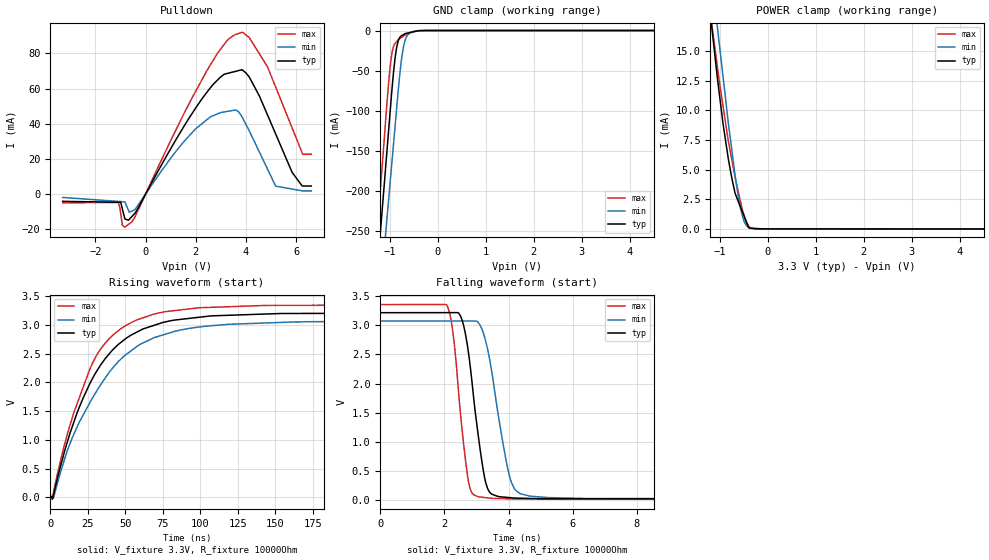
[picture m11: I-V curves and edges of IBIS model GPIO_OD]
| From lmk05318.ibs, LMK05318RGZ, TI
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|   GPIO_OD Model
[Model]   GPIO_OD
Model_type   I/O_open_drain
Polarity   Non-Inverting
Enable   Active-Low
Vinl = 0.6
Vinh = 1.1
Vmeas = 1.65
Vref = 3.3
Cref = 2pF
Rref = 10000
|   typ   min   max
C_comp   1.6827E-12   1.6616E-12  1.6834E-12
| Where nom  PVT is Nominal Process, 3.3V, 27C
|   Fast PVT is Strong Process,  3.45V, -40C
|   Slow PVT is Weak Process,   3.15V, 125C
[Model spec]
|subparameter
Vinl   0.6   0.57   0.63
Vinh   1.1   1.05   1.15
[Voltage Range]   3.3   3.15   3.45
|Junction Temperature
[Temperature Range]   27   125   -40
[Pullup Reference]   3.3   3.15   3.45
[Pulldown Reference]   -0   -0   0
[Power Clamp Reference]   3.3   3.15   3.45
[GND Clamp Reference]   0   0   0
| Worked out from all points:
|   slope of the pulldown table from 0 to 0.495 V, typ, clamps not added: 38.1 ohm
|   GND clamp passes 1 mA (typ) near -0.47 V on its own axis
|   POWER clamp passes 1 mA (typ) near -0.49 V on its own axis
|   falling waveform, V_fixture 3.3V, R_fixture 10000Ohm: 20-80 % time 434ps typ, 549ps min, 352ps max; typ from 3.22 V to 0.012 V
|   rising waveform, V_fixture 3.3V, R_fixture 10000Ohm: 20-80 % time 33.9ns typ, 40.2ns min, 29.5ns max; typ from 0.012 V to 3.22 V
[Pulldown]
|   Voltage   I(typ)   I(min)   I(max)
-3.3V     -4.119mA   -1.898mA   -4.984mA
-1.087V   -4.62mA    -4.15mA    -4.728mA
-922.7mV  -8.493mA   -4.317mA   -17.77mA
-825mV    -14.1mA    -4.417mA   -18.79mA
-542.2mV  -12.7mA    -9.677mA   -15.7mA
2.003V    49.12mA    37.22mA    58.69mA
3.232V    68.5mA     46.95mA    87.07mA
3.841V    70.7mA     43.86mA    91.96mA
4.855V    45mA       14.24mA    72.37mA
5.18V     34.18mA    4.53mA     60.85mA
6.259V    4.588mA    1.802mA    22.62mA
6.6V      4.588mA    1.802mA    22.62mA
[GND Clamp]
|   Voltage   I(typ)   I(min)   I(max)
-3.3V     -1.815A    -1.777A    -1.852A
-1.266V   -302.4mA   -374.5mA   -252.1mA
-1.049V   -141.6mA   -226.7mA   -81.69mA
-973mV    -85.15mA   -174.8mA   -34.59mA
-929.8mV  -55.65mA   -145.5mA   -20.87mA
-859.1mV  -21.04mA   -97.37mA   -13.83mA
-825mV    -12.6mA    -74.12mA   -11.44mA
-757.1mV  -6.495mA   -35.86mA   -8.622mA
-683.6mV  -3.842mA   -12.56mA   -5.839mA
-579mV    -2.479mA   -2.982mA   -2.654mA
-229mV    -6.598uA   -15.66uA   -34.65uA
6.6V      0A         0A         0A
[POWER Clamp]
|   Voltage   I(typ)   I(min)   I(max)
-3.3V     104.9mA    103mA      109.7mA
-1.21V    18.54mA    22.75mA    18.47mA
-1.137V   15.83mA    20.01mA    16.24mA
-1.054V   12.78mA    17.08mA    13.74mA
-934.9mV  8.882mA    12.86mA    10.37mA
-825mV    5.929mA    8.968mA    7.425mA
-683.6mV  3.01mA     4.53mA     4.376mA
-628.7mV  2.447mA    3.048mA    3.351mA
-535.3mV  1.49mA     1.138mA    1.694mA
-400.8mV  110.9uA    120.1uA    263.7uA
-118mV    10.15uA    8.394uA    9.963uA
6.6V      0A         0A         0A
[Ramp]
R_load = 10000
|   typ   min   max
dV/dt_r   1.92339/3.39818e-08   1.83659/4.02712e-08   2.00774/2.94956e-08
dV/dt_f   1.9234/4.32954e-10   1.83659/5.48867e-10   2.00775/3.51466e-10
[Falling Waveform]
V_fixture = 3.3V
V_fixture_min = 3.15V
V_fixture_max = 3.45V
R_fixture = 10000Ohm
C_fixture = 0F
|   Time   V(typ)   V(min)   V(max)
0s        3.218V     3.076V     3.357V
2.074ns   3.219V     3.076V     3.349V
2.256ns   3.219V     3.076V     2.921V
2.451ns   3.21V      3.076V     1.789V
2.806ns   2.295V     3.076V     188mV
3.19ns    585.5mV    2.907V     45.67mV
3.466ns   106.6mV    2.242V     29.04mV
4.094ns   37.16mV    296.4mV    19.16mV
5.243ns   20.73mV    41.04mV    17.97mV
100ns     12.45mV    14.67mV    11.11mV
[Rising Waveform]
V_fixture = 3.3V
V_fixture_min = 3.15V
V_fixture_max = 3.45V
R_fixture = 10000Ohm
C_fixture = 0F
|   Time   V(typ)   V(min)   V(max)
0s        12.45mV    14.67mV    11.11mV
1.19ns    -8.932mV   11mV       -36.63mV
2.086ns   34.48mV    -14.98mV   82.45mV
15.34ns   1.281V     1.076V     1.444V
30.81ns   2.191V     1.845V     2.471V
49.3ns    2.744V     2.463V     2.976V
69.1ns    2.994V     2.779V     3.19V
102.2ns   3.144V     2.975V     3.304V
163.9ns   3.201V     3.054V     3.343V
500ns     3.218V     3.076V     3.357V
